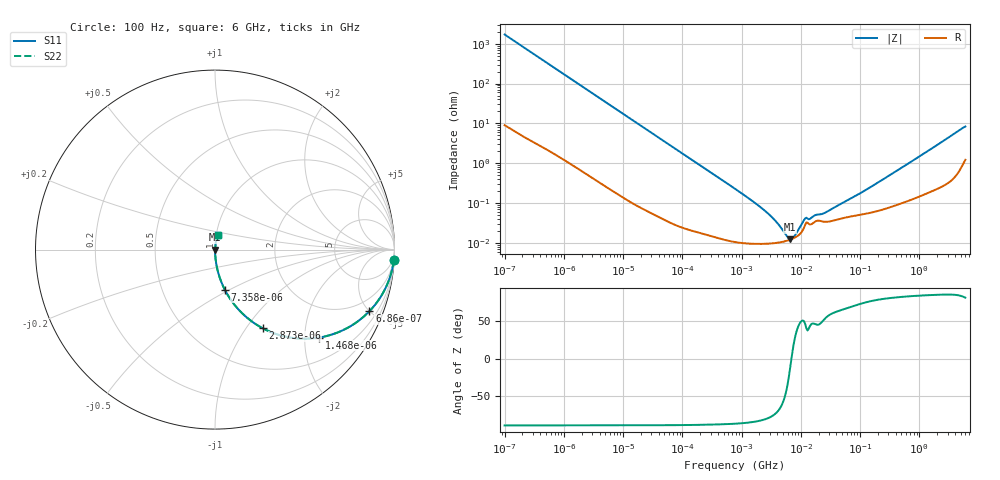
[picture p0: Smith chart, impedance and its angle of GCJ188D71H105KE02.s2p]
!Murata Part Number: GCJ188D71H105KE02
!These Parameters are Measured in Series Mode Connection
!Data Generated on Mar 13, 2026
!  o--ll--o
!Port1  Port2
!  o------o
!Operation Temp=25[degC], DC Bias Voltage=0[V]
!Freq. Start=100[Hz] Stop=6[GHz] 401[Steps]
# Hz S RI R 50
!Freq.(Hz) S11(Real) S11(Imag) S21(Real) S21(Imag) S12(Real) S12(Imag) S22(Real) S22(Imag)
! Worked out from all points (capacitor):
!   401 points, 100 Hz to 6 GHz, reference 50 ohm
!   read as one part in series: C = 932 nF near 109 Hz
!   lowest |Z| = 12.3 mohm at 6.644 MHz (marker M1)
!   series resonance near 6.953 MHz, so ESL is about 560 pH
!   S11 on the Smith chart (normalised r, x): 100 Hz: 1, -34; 686 Hz: 1.03, -5.01; 1.468 kHz: 1.02, -2.35; 2.873 kHz: 1.01, -1.20; 7.358 kHz: 1.00, -0.47; 6 GHz: 1.02, +0.16
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100  0.9963 -0.0584  0.00374 0.0584  0.00374 0.0584  0.9963 -0.0584
268  0.9752 -0.1526  0.0248 0.1526  0.0248 0.1526  0.9752 -0.1526
686  0.8607 -0.3429  0.1393 0.3429  0.1393 0.3429  0.8607 -0.3429
981  0.7529 -0.4278  0.2471 0.4278  0.2471 0.4278  0.7529 -0.4278
1468  0.5788 -0.4901  0.4212 0.4901  0.4212 0.4901  0.5788 -0.4901
2008  0.4252 -0.4907  0.5748 0.4907  0.5748 0.4907  0.4252 -0.4907
2873  0.2672 -0.4388  0.7328 0.4388  0.7328 0.4388  0.2672 -0.4388
4496  0.1311 -0.3337  0.8689 0.3337  0.8689 0.3337  0.1311 -0.3337
7358  0.0543 -0.2227  0.9457 0.2227  0.9457 0.2227  0.0543 -0.2227
15752  0.013 -0.109  0.987 0.109  0.987 0.109  0.013 -0.109
40335  0.00232 -0.0433  0.9977 0.0433  0.9977 0.0433  0.00232 -0.0433
774597  0.00011 -0.00227  0.9999 0.00227  0.9999 0.00227  0.00011 -0.00227
2837864  9.56e-05 -0.000526  0.9999 0.000526  0.9999 0.000526  9.56e-05 -0.000526
4060267  0.000101 -0.000291  0.9999 0.000291  0.9999 0.000291  0.000101 -0.000291
5809218  0.000112 -9.39e-05  0.9999 9.39e-05  0.9999 9.39e-05  0.000112 -9.39e-05
6644369  0.00012 -2.37e-05  0.9999 2.37e-05  0.9999 2.37e-05  0.00012 -2.37e-05
7947587  0.000135 7.1e-05  0.9999 -7.1e-05  0.9999 -7.1e-05  0.000135 7.1e-05
1.137099e7  0.000243 0.000287  0.9998 -0.000287  0.9998 -0.000287  0.000243 0.000287
1.555665e7  0.000302 0.000321  0.9997 -0.000321  0.9997 -0.000321  0.000302 0.000321
2.784235e7  0.000338 0.000505  0.9997 -0.000505  0.9997 -0.000505  0.000338 0.000505
3.124326e8  0.000793 0.00486  0.9992 -0.00486  0.9992 -0.00486  0.000793 0.00486
6e9  0.0185 0.08  0.9815 -0.08  0.9815 -0.08  0.0185 0.08
